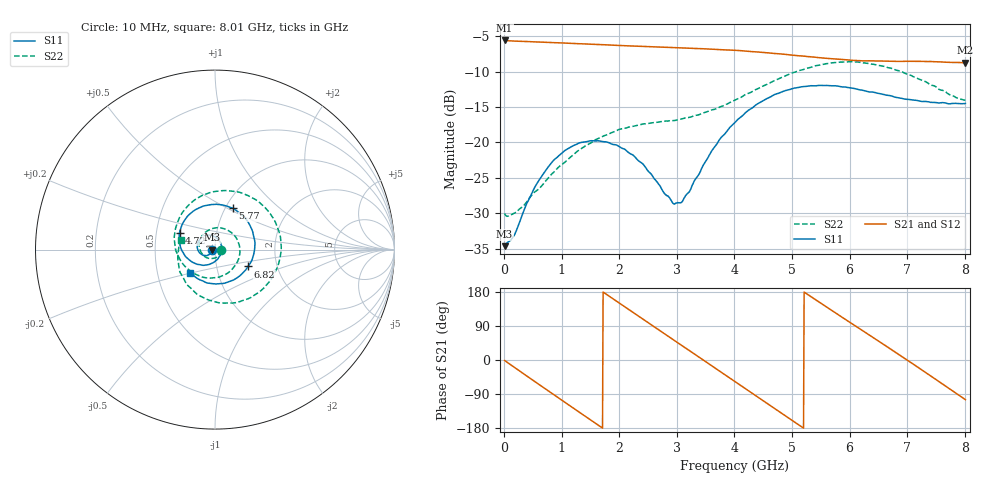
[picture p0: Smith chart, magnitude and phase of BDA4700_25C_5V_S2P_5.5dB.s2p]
!Agilent Technologies,E5071B,MY42404982,A.09.10
!Date: Mon Oct 20 13:28:40 2025
!Data & Calibration Information:
!Freq	S11:SOLT2(ON)	S21:SOLT2(ON)	S12:SOLT2(ON)	S22:SOLT2(ON)
# Hz S RI R 50
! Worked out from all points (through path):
!   801 points, 10 MHz to 8.01 GHz, reference 50 ohm
!   highest |S21| = -5.62 dB at 10 MHz (marker M1); lowest = -8.8 dB at 8.01 GHz (marker M2)
!   group delay of S21, straight-line fit = 285 ps
!   lowest |S11| = -34.6 dB at 10 MHz (marker M3), VSWR 1.04, Z = 48.2 - j0.109 ohm
!   |S11| at or under -10 dB: start of sweep to end of sweep
!   |S22| runs from -30.4 to -8.6 dB; largest |S21 - S12| = 0.004
!   S11 on the Smith chart (normalised r, x): 10 MHz: 0.96, -0.00; 4.72 GHz: 0.66, +0.13; 5.77 GHz: 1.08, +0.53; 6.82 GHz: 1.42, -0.28; 8.01 GHz: 0.73, -0.19
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1e7  -0.0185 -0.00113  0.5235 -0.0113  0.5234 -0.0117  0.0315 -0.00259
3.3e8  -0.0247 -0.0203  0.4206 -0.2982  0.4206 -0.2987  0.022 -0.0279
7.1e8  -0.0525 -0.0336  0.129 -0.492  0.1285 -0.4923  -0.0163 -0.0502
1.02e9  -0.0827 -0.021  -0.1536 -0.4783  -0.1538 -0.4788  -0.0614 -0.0351
1.35e9  -0.0992 0.0139  -0.3921 -0.3037  -0.3925 -0.3039  -0.088 0.0226
1.64e9  -0.0898 0.0501  -0.4859 -0.0646  -0.486 -0.0648  -0.0665 0.0836
1.93e9  -0.06 0.0753  -0.4473 0.1851  -0.4475 0.185  -0.00242 0.1199
2.32e9  -0.00836 0.0747  -0.2182 0.4239  -0.2182 0.424  0.0979 0.0891
2.68e9  0.0286 0.0423  0.08 0.4641  0.0802 0.464  0.1388 -0.00857
3.04e9  0.036 -0.0105  0.3398 0.3173  0.3384 0.3182  0.0957 -0.1092
3.36e9  0.0107 -0.0566  0.452 0.0807  0.4526 0.0806  0.00604 -0.156
3.67e9  -0.0421 -0.0845  0.4206 -0.1688  0.4204 -0.17  -0.096 -0.143
4.01e9  -0.1167 -0.0744  0.242 -0.3745  0.2423 -0.3744  -0.1867 -0.0692
4.36e9  -0.1816 -0.0104  -0.0255 -0.4349  -0.026 -0.4354  -0.2269 0.0602
4.72e9  -0.1976 0.0951  -0.2756 -0.321  -0.2752 -0.3218  -0.1804 0.2083
5.35e9  -0.0549 0.2449  -0.3869 0.1037  -0.3873 0.103  0.1034 0.3244
5.77e9  0.0984 0.2304  -0.2097 0.3255  -0.2091 0.3258  0.3026 0.2064
6.2e9  0.2038 0.1153  0.0643 0.3709  0.0679 0.3714  0.3646 -0.0327
6.68e9  0.2082 -0.0517  0.3167 0.1985  0.3175 0.1977  0.2201 -0.2533
6.82e9  0.1846 -0.0942  0.3548 0.1154  0.3554 0.1137  0.1511 -0.2854
7.32e9  0.0538 -0.187  0.3121 -0.2027  0.3118 -0.2039  -0.0993 -0.2491
8.01e9  -0.1385 -0.1276  -0.0922 -0.3528  -0.0923 -0.353  -0.1917 0.0519
